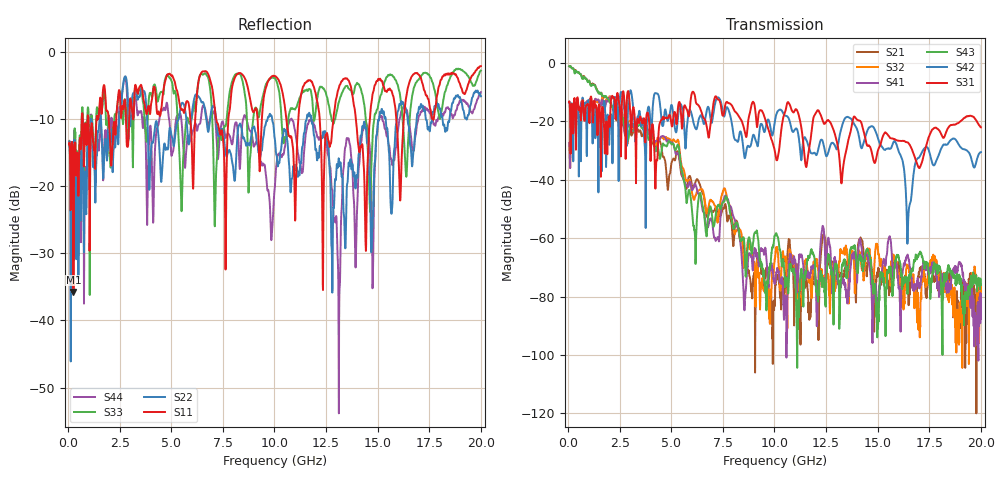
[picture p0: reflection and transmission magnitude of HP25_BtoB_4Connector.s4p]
# MHz S MA R 50.00
! FREQ  S11  S12  S13  S14
!  S21  S22  S23  S24
!  S31  S32  S33  S34
!  S41  S42  S43  S44
!  MAG  ANG  MAG  ANG  MAG  ANG  MAG  ANG
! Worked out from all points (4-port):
!   1996 points, 50 MHz to 20 GHz, reference 50 ohm
!   strongest paths, dB at 50 MHz, 5.04 GHz, 10.03 GHz, 15.02 GHz, 20 GHz:
!     S31: -13.4, -21.7, -30.8, -29.8, -22.0
!     S42: -13.5, -14.8, -19.5, -26.0, -30.5
!     S43: -1.1, -27.8, -59.1, -89.6, -75.8
!     S41: -27.4, -27.2, -75.5, -82.3, -87.5
!     S32: -27.4, -27.0, -66.6, -64.3, -78.7
!     S21: -1.1, -33.6, -79.1, -71.9, -85.5
!   lowest |S11| = -35.8 dB at 260 MHz (marker M1), VSWR 1.03, Z = 49.4 + j1.49 ohm
!   |S11| at or under -10 dB: start of sweep to 664.8 MHz; 12.19 GHz to 12.86 GHz (667.9 MHz wide, 5.33 % of centre); 13.94 GHz to 14.62 GHz (681.8 MHz wide, 4.77 % of centre)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
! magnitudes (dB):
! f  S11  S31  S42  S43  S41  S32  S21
! 50 MHz  -13.8  -13.4  -13.5  -1.1  -27.4  -27.4  -1.1
! 260 MHz  -35.8  -18.7  -22.3  -2.0  -19.1  -19.0  -2.0
! 5.28 GHz  -5.8  -19.3  -22.0  -28.4  -31.0  -26.6  -30.3
! 9.6 GHz  -5.2  -20.5  -21.1  -79.7  -66.3  -77.4  -70.9
! 14.75 GHz  -6.4  -31.8  -21.8  -75.8  -95.9  -74.8  -73.7
! 16.48 GHz  -5.2  -27.4  -53.3  -75.8  -66.6  -69.4  -79.3
! 20 GHz  -2.2  -22.0  -30.5  -75.8  -87.5  -78.7  -85.5
